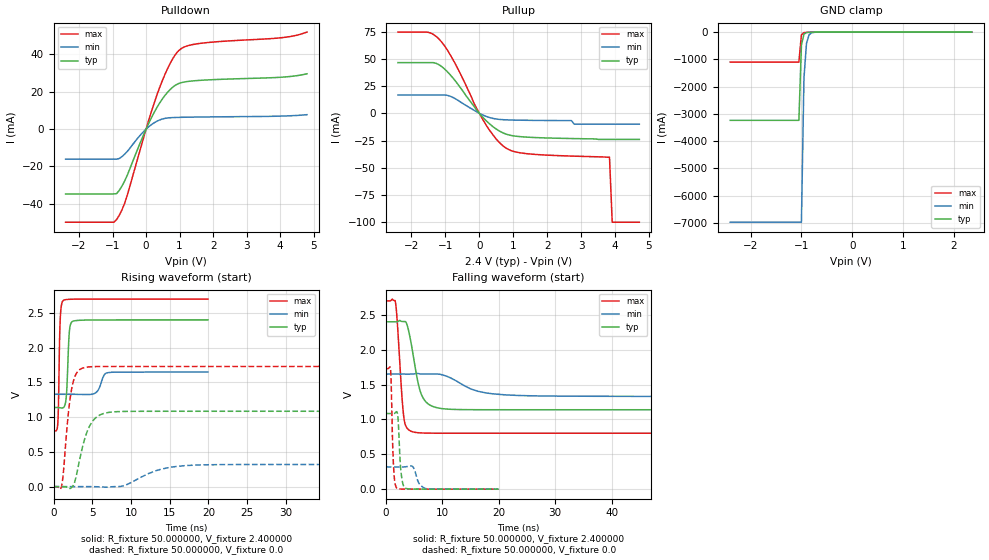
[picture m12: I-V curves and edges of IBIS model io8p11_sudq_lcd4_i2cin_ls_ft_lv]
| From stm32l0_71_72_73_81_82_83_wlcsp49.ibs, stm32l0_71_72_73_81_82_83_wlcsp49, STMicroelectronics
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|   Model io8p11_sudq_lcd4_i2cin_ls_ft_lv
[Model]  io8p11_sudq_lcd4_i2cin_ls_ft_lv
Model_type I/O
Polarity   Non-Inverting
Enable   Active-Low
Vinl =   0.720000V
Vinh =   1.680000V
Vmeas =  1.200000V
Cref =   50.000000pF
Rref =   100.000000M
Vref =   0.0V
C_comp   2.470900pF   2.435200pF   2.508800pF
[Temperature Range]   25.000000   0.125000k   -40.000000
[Pullup Reference]   2.400000V   1.650000V   2.700000V
[Pulldown Reference]   0.0V   0.0V   0.0V
[POWER Clamp Reference]   2.400000V   1.650000V   2.700000V
[GND Clamp Reference]   0.0V   0.0V   0.0V
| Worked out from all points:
|   slope of the pulldown table from 0 to 0.36 V, typ, clamps not added: 28.5 ohm
|   slope of the pullup table from 0 to 0.36 V, typ, clamps not added: 32.2 ohm
|   GND clamp passes 1 mA (typ) near -0.64 V on its own axis
|   rising waveform, R_fixture 50.000000, V_fixture 2.400000: 20-80 % time 284ps typ, 659ps min, 195ps max; typ from 1.14 V to 2.4 V
|   rising waveform, R_fixture 50.000000, V_fixture 0.0: 20-80 % time 1.58ns typ, 3.96ns min, 926ps max; typ from 0 V to 1.08 V
|   falling waveform, R_fixture 50.000000, V_fixture 2.400000: 20-80 % time 1.8ns typ, 5.23ns min, 905ps max; typ from 2.4 V to 1.14 V
|   falling waveform, R_fixture 50.000000, V_fixture 0.0: 20-80 % time 465ps typ, 886ps min, 363ps max; typ from 1.08 V to 0 V
[Pulldown]
|Voltage   I(typ)   I(min)   I(max)
-2.4V     -34.7mA    -16.06mA   -49.82mA
-960mV    -34.7mA    -16.06mA   -49.82mA
-880mV    -34.55mA   -16.06mA   -48.46mA
-720mV    -30.52mA   -14.74mA   -43.28mA
-560mV    -24.65mA   -11.94mA   -35.33mA
0V        326fA      0A         16fA
400mV     13.84mA    4.882mA    22.03mA
720mV     21.25mA    6.107mA    35.26mA
1.04V     24.82mA    6.324mA    43.03mA
1.6V      26.11mA    6.486mA    45.88mA
4V        27.76mA    6.965mA    48.87mA
4.8V      29.63mA    7.736mA    51.96mA
[Pullup]
|Voltage   I(typ)   I(min)   I(max)
-2.4V     46.57mA    16.84mA    74.62mA
-1.52V    46.57mA    16.84mA    74.5mA
-1.2V     44.83mA    16.84mA    68.61mA
-720mV    30.24mA    13.64mA    46.11mA
-160mV    6.586mA    2.887mA    9.467mA
160mV     -5.477mA   -2.317mA   -8.695mA
480mV     -14.04mA   -5.139mA   -22.91mA
800mV     -19.2mA    -6.004mA   -32.18mA
1.52V     -22.07mA   -6.444mA   -37.42mA
3.84V     -24mA      -10mA      -40.3mA
3.92V     -24mA      -10mA      -100mA
4.72V     -24mA      -10mA      -100mA
[GND_clamp]
|Voltage   I(typ)   I(min)   I(max)
-2.4V     -3.237A    -6.973A    -1.1A
-1.05V    -3.237A    -6.973A    -1.1A
-1V       -475.5mA   -6.973A    -104.1mA
-950mV    -76.08mA   -1.682A    -18.44mA
-900mV    -16.57mA   -411.5mA   -9.263mA
-850mV    -6.62mA    -103.7mA   -6.764mA
-800mV    -4.092mA   -27.93mA   -4.994mA
-600mV    -527.6uA   -834.2uA   -509uA
2.35V     0A         0A         0A
[POWER_clamp]
|Voltage   I(typ)   I(min)   I(max)
-2.4V     0A         0A         0A
0V        0A         0A         0A
[Ramp]
| variable   typ   min   max
dV/dt_r  0.65070/1.58160n   0.19118/3.95450n   1.03800/0.92304n
dV/dt_f  0.75690/1.79566n   0.18912/5.22749n   1.13815/0.90300n
R_load = 50.000000
[Rising Waveform]
R_fixture= 50.000000
V_fixture= 2.400000
V_fixture_min= 1.650000
V_fixture_max= 2.700000
|time   V(typ)   V(min)   V(max)
0s        1.139V     1.329V     802mV
560.6ps   1.138V     1.329V     921.6mV
840.8ps   1.135V     1.329V     2.347V
1.241ns   1.135V     1.329V     2.678V
1.642ns   1.288V     1.329V     2.693V
2.082ns   2.27V      1.329V     2.697V
2.442ns   2.378V     1.329V     2.698V
5.365ns   2.399V     1.345V     2.7V
7.007ns   2.4V       1.64V      2.7V
19.94ns   2.4V       1.65V      2.7V
[Rising Waveform]
R_fixture= 50.000000
V_fixture= 0.0
V_fixture_min= 0.0
V_fixture_max= 0.0
|time   V(typ)   V(min)   V(max)
0s        -2.924uV   3.933uV    227uV
1.001ns   109.6uV    1.235uV    -13.29mV
1.251ns   -712.6uV   -1.604uV   176mV
1.877ns   -10.77mV   -4.809uV   1.016V
2.377ns   -7.649mV   10.58uV    1.428V
4.004ns   679.5mV    81.75uV    1.714V
5.38ns    984.1mV    -1.596mV   1.728V
8.008ns   1.078V     -449.3uV   1.73V
17.14ns   1.085V     303.6mV    1.73V
62.31ns   1.085V     318.6mV    1.73V
[Falling Waveform]
R_fixture= 50.000000
V_fixture= 2.400000
V_fixture_min= 1.650000
V_fixture_max= 2.700000
|time   V(typ)   V(min)   V(max)
0s        2.4V       1.65V      2.7V
1.627ns   2.4V       1.65V      2.706V
2.002ns   2.401V     1.65V      2.423V
3.128ns   2.404V     1.65V      1.066V
3.754ns   2.355V     1.65V      874.8mV
4.505ns   2.08V      1.65V      829.5mV
6.381ns   1.341V     1.652V     805.8mV
9.259ns   1.164V     1.65V      802.4mV
21.27ns   1.139V     1.351V     802mV
62.31ns   1.139V     1.329V     802mV
[Falling Waveform]
R_fixture= 50.000000
V_fixture= 0.0
V_fixture_min= 0.0
V_fixture_max= 0.0
|time   V(typ)   V(min)   V(max)
0s        1.085V     318.6mV    1.73V
840.8ps   1.085V     318.6mV    1.706V
1.361ns   1.084V     318.6mV    328.5mV
1.922ns   1.111V     318.6mV    15.07mV
2.162ns   1.005V     318.6mV    4.668mV
2.683ns   248.6mV    318.3mV    2.215mV
3.323ns   21.81mV    319.3mV    1.429mV
4.725ns   1.832mV    325.3mV    598.7uV
7.207ns   460.7uV    6.609mV    276uV
19.94ns   -2.924uV   3.933uV    227uV
